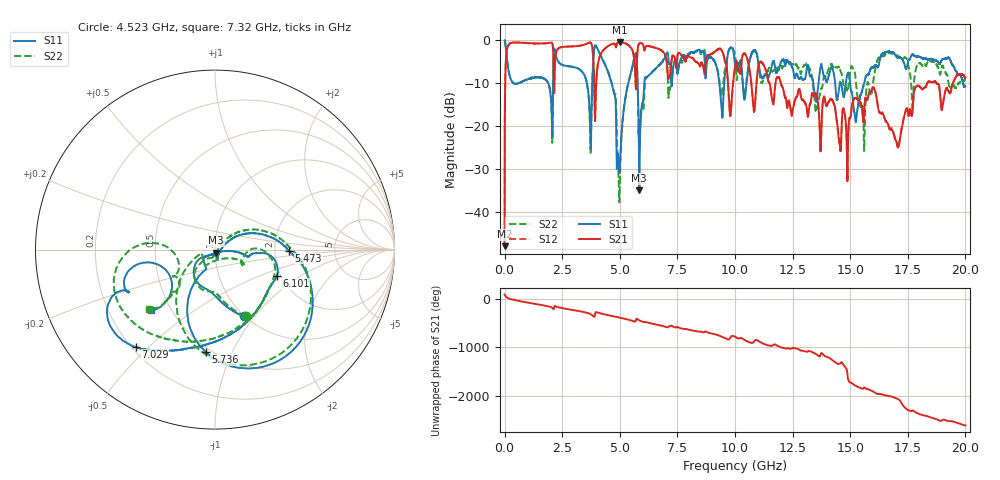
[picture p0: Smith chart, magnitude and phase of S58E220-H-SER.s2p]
!{S58E220}
!Johanson Technology Inc.
!www.johansontechnology.com
!Test Board Conditions:
!Substrate Type  RO4350B
!Substrate Thickness  60 mil
!Substrate Dk  3.66
!TL Type: GCPW
!TL Trace Width  115 mil
!TL Gap  52 mil
!Electrode orientation  Horizontal
!DUT TOPOLOGY	SERIES
!Mounting Pad LxW  55x428 mil
! Created Wed Apr 14 11:29:40 2021
# mhz S ma R 50
! 2 Port Network Data from SP1.SP block
! freq  magS11  angS11  magS21  angS21  magS12  angS12  magS22  angS22
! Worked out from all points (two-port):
!   20001 points, 300 kHz to 20 GHz, reference 50 ohm
!   highest |S21| = -0.41 dB at 4.988 GHz (marker M1); lowest = -47.9 dB at 300 kHz (marker M2)
!   |S21| within 3 dB of the highest: 70.84 MHz to 2.113 GHz (2.043 GHz wide, 187 % of centre); 2.215 GHz to 3.839 GHz (1.624 GHz wide, 53.7 % of centre)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
!   lowest |S11| = -34.9 dB at 5.846 GHz (marker M3), VSWR 1.04, Z = 50.6 - j1.72 ohm
!   |S11| at or under -10 dB: 4.647 GHz to 5.364 GHz (717.5 MHz wide, 14.3 % of centre); 5.777 GHz to 6.065 GHz (288.5 MHz wide, 4.87 % of centre); 15 GHz to 15.61 GHz (610 MHz wide, 3.99 % of centre)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
!   |S22| runs from -37.7 to 0.0 dB; largest |S21 - S12| = 0.01
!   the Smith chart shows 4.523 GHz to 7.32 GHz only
!   S11 on the Smith chart (normalised r, x): 4.523 GHz: 0.99, -0.89; 5.473 GHz: 2.40, -0.03; 5.736 GHz: 0.47, -0.79; 6.101 GHz: 1.90, -0.65; 7.029 GHz: 0.21, -0.46; 7.32 GHz: 0.39, -0.35
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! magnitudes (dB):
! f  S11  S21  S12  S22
! 300 kHz  0.0  -47.9  -47.8  0.0
! 103.3 MHz  -4.4  -2.0  -2.1  -4.4
! 199.3 MHz  -7.9  -0.9  -0.9  -7.8
! 3.334 GHz  -7.1  -1.1  -1.1  -7.1
! 3.698 GHz  -17.7  -0.5  -0.5  -18.0
! 3.951 GHz  -1.1  -13.7  -13.7  -1.2
! 4.523 GHz  -7.8  -1.2  -1.2  -7.8
! 4.988 GHz  -30.3  -0.4  -0.4  -36.6
! 5.473 GHz  -7.7  -1.6  -1.6  -7.8
! 5.736 GHz  -4.9  -6.0  -6.0  -5.4
! 5.846 GHz  -34.9  -0.7  -0.7  -24.5
! 6.101 GHz  -8.5  -1.8  -1.8  -9.2
! 6.667 GHz  -5.9  -1.9  -1.9  -6.0
! 7.029 GHz  -3.1  -4.8  -4.8  -4.3
! 7.32 GHz  -6.2  -3.6  -3.5  -6.1
! 9.428 GHz  -16.6  -2.5  -2.5  -12.7
! 10 GHz  -5.6  -6.5  -6.5  -3.4
! 13.33 GHz  -8.5  -12.7  -12.6  -8.2
! 15.11 GHz  -13.5  -14.3  -14.3  -6.5
! 15.56 GHz  -10.9  -18.3  -18.3  -16.3
! 16.67 GHz  -2.6  -20.1  -19.8  -2.8
! 20 GHz  -10.7  -8.7  -8.7  -8.7
